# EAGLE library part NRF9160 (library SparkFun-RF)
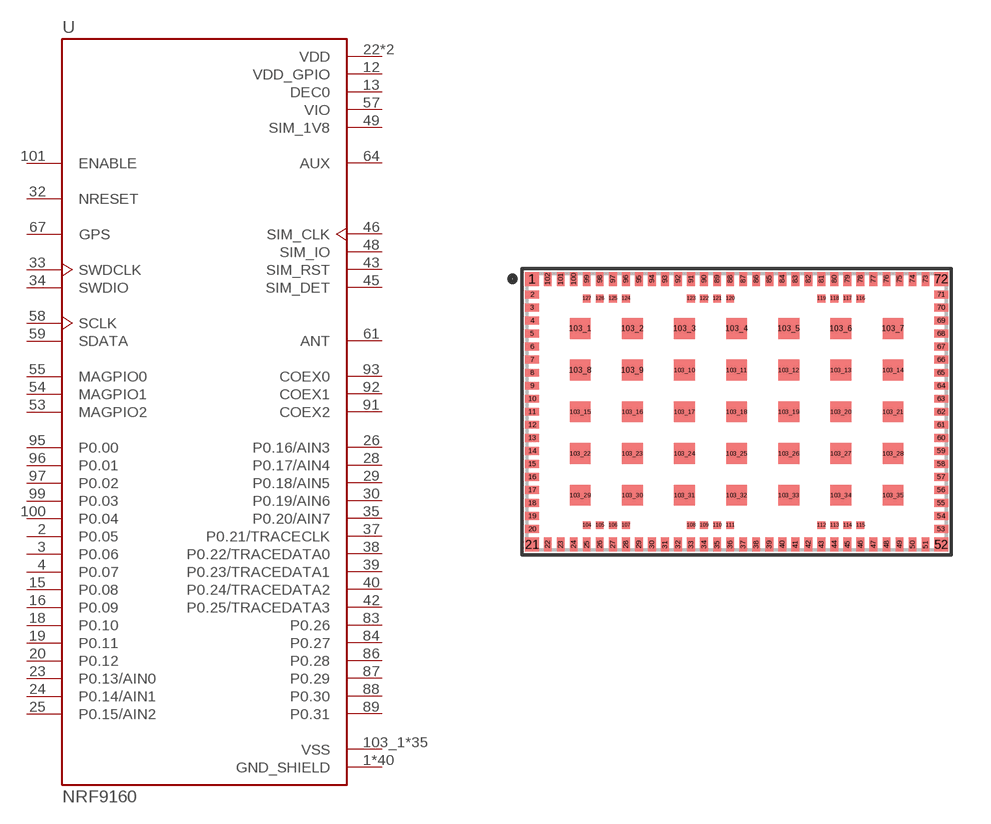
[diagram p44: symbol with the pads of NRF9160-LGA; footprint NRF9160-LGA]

Designator prefix -

## NRF9160 (PROD_ID: IC-15418; VALUE: NRF9160-SICA-R)  [NRF9160-LGA]
1  GND_SHIELD  pwr
2  P0.05
3  P0.06
4  P0.07
5  GND_SHIELD  pwr
6  GND_SHIELD  pwr
7  GND_SHIELD  pwr
8  GND_SHIELD  pwr
9  GND_SHIELD  pwr
11  GND_SHIELD  pwr
12  VDD_GPIO  pwr
13  DEC0  pwr
14  GND_SHIELD  pwr
15  P0.08
16  P0.09
17  GND_SHIELD  pwr
18  P0.10
19  P0.11
20  P0.12
21  GND_SHIELD  pwr
22  VDD  pwr
23  P0.13/AIN0
24  P0.14/AIN1
25  P0.15/AIN2
26  P0.16/AIN3
27  GND_SHIELD  pwr
28  P0.17/AIN4
29  P0.18/AIN5
30  P0.19/AIN6
31  GND_SHIELD  pwr
32  NRESET  in
33  SWDCLK  in
34  SWDIO
35  P0.20/AIN7
36  GND_SHIELD  pwr
37  P0.21/TRACECLK
38  P0.22/TRACEDATA0
39  P0.23/TRACEDATA1
40  P0.24/TRACEDATA2
41  GND_SHIELD  pwr
42  P0.25/TRACEDATA3
43  SIM_RST
44  GND_SHIELD  pwr
45  SIM_DET
46  SIM_CLK
47  GND_SHIELD  pwr
48  SIM_IO
49  SIM_1V8  pwr
50  GND_SHIELD  pwr
52  GND_SHIELD  pwr
53  MAGPIO2
54  MAGPIO1
55  MAGPIO0
56  GND_SHIELD  pwr
57  VIO  pwr
58  SCLK
59  SDATA
60  GND_SHIELD  pwr
61  ANT
62  GND_SHIELD  pwr
63  GND_SHIELD  pwr
64  AUX  out
65  GND_SHIELD  pwr
66  GND_SHIELD  pwr
67  GPS  in
68  GND_SHIELD  pwr
69  GND_SHIELD  pwr
72  GND_SHIELD  pwr
74  GND_SHIELD  pwr
75  GND_SHIELD  pwr
76  GND_SHIELD  pwr
77  GND_SHIELD  pwr
78  GND_SHIELD  pwr
79  GND_SHIELD  pwr
80  GND_SHIELD  pwr
81  GND_SHIELD  pwr
82  GND_SHIELD  pwr
83  P0.26
84  P0.27
85  GND_SHIELD  pwr
86  P0.28
87  P0.29
88  P0.30
89  P0.31
90  GND_SHIELD  pwr
91  COEX2
92  COEX1
93  COEX0
94  GND_SHIELD  pwr
95  P0.00
96  P0.01
97  P0.02
98  GND_SHIELD  pwr
99  P0.03
100  P0.04
101  ENABLE  in
102  VDD  pwr
103_1  VSS  pwr
103_2  VSS  pwr
103_3  VSS  pwr
103_4  VSS  pwr
103_5  VSS  pwr
103_6  VSS  pwr
103_7  VSS  pwr
103_8  VSS  pwr
103_9  VSS  pwr
103_10  VSS  pwr
103_11  VSS  pwr
103_12  VSS  pwr
103_13  VSS  pwr
103_14  VSS  pwr
103_15  VSS  pwr
103_16  VSS  pwr
103_17  VSS  pwr
103_18  VSS  pwr
103_19  VSS  pwr
103_20  VSS  pwr
103_21  VSS  pwr
103_22  VSS  pwr
103_23  VSS  pwr
103_24  VSS  pwr
103_25  VSS  pwr
103_26  VSS  pwr
103_27  VSS  pwr
103_28  VSS  pwr
103_29  VSS  pwr
103_30  VSS  pwr
103_31  VSS  pwr
103_32  VSS  pwr
103_33  VSS  pwr
103_34  VSS  pwr
103_35  VSS  pwr

## Footprint NRF9160-LGA (pad centres in mm)
smd 0.54 x 0.54: 1 -7.845,5.095; 21 -7.845,-5.095; 52 7.845,-5.095; 72 7.845,5.095
smd 0.54 x 0.3: 2 -7.845,4.5; 3 -7.845,4; 4 -7.845,3.5; 5 -7.845,3; 6 -7.845,2.5; 7 -7.845,2; 8 -7.845,1.5; 9 -7.845,1; 10 -7.845,0.5; 11 -7.845,0; 12 -7.845,-0.5; 13 -7.845,-1; 14 -7.845,-1.5; 15 -7.845,-2; 16 -7.845,-2.5; 17 -7.845,-3; 18 -7.845,-3.5; 19 -7.845,-4; 20 -7.845,-4.5; 53 7.845,-4.5; 54 7.845,-4; 55 7.845,-3.5; 56 7.845,-3; 57 7.845,-2.5; 58 7.845,-2; 59 7.845,-1.5; 60 7.845,-1; 61 7.845,-0.5; 62 7.845,0; 63 7.845,0.5; 64 7.845,1; 65 7.845,1.5; 66 7.845,2; 67 7.845,2.5; 68 7.845,3; 69 7.845,3.5; 70 7.845,4; 71 7.845,4.5
smd 0.3 x 0.54: 22 -7.25,-5.095; 23 -6.75,-5.095; 24 -6.25,-5.095; 25 -5.75,-5.095; 26 -5.25,-5.095; 27 -4.75,-5.095; 28 -4.25,-5.095; 29 -3.75,-5.095; 30 -3.25,-5.095; 31 -2.75,-5.095; 32 -2.25,-5.095; 33 -1.75,-5.095; 34 -1.25,-5.095; 35 -0.75,-5.095; 36 -0.25,-5.095; 37 0.25,-5.095; 38 0.75,-5.095; 39 1.25,-5.095; 40 1.75,-5.095; 41 2.25,-5.095; 42 2.75,-5.095; 43 3.25,-5.095; 44 3.75,-5.095; 45 4.25,-5.095; 46 4.75,-5.095; 47 5.25,-5.095; 48 5.75,-5.095; 49 6.25,-5.095; 50 6.75,-5.095; 51 7.25,-5.095; 73 7.25,5.095; 74 6.75,5.095; 75 6.25,5.095; 76 5.75,5.095; 77 5.25,5.095; 78 4.75,5.095; 79 4.25,5.095; 80 3.75,5.095; 81 3.25,5.095; 82 2.75,5.095; 83 2.25,5.095; 84 1.75,5.095; 85 1.25,5.095; 86 0.75,5.095; 87 0.25,5.095; 88 -0.25,5.095; 89 -0.75,5.095; 90 -1.25,5.095; 91 -1.75,5.095; 92 -2.25,5.095; 93 -2.75,5.095; 94 -3.25,5.095; 95 -3.75,5.095; 96 -4.25,5.095; 97 -4.75,5.095; 98 -5.25,5.095; 99 -5.75,5.095; 100 -6.25,5.095; 101 -6.75,5.095; 102 -7.25,5.095
smd 0.8 x 0.8: 103_1 -6,3.2; 103_2 -4,3.2; 103_3 -2,3.2; 103_4 0,3.2; 103_5 2,3.2; 103_6 4,3.2; 103_7 6,3.2; 103_8 -6,1.6; 103_9 -4,1.6; 103_10 -2,1.6; 103_11 0,1.6; 103_12 2,1.6; 103_13 4,1.6; 103_14 6,1.6; 103_15 -6,0; 103_16 -4,0; 103_17 -2,0; 103_18 0,0; 103_19 2,0; 103_20 4,0; 103_21 6,0; 103_22 -6,-1.6; 103_23 -4,-1.6; 103_24 -2,-1.6; 103_25 0,-1.6; 103_26 2,-1.6; 103_27 4,-1.6; 103_28 6,-1.6; 103_29 -6,-3.2; 103_30 -4,-3.2; 103_31 -2,-3.2; 103_32 0,-3.2; 103_33 2,-3.2; 103_34 4,-3.2; 103_35 6,-3.2
smd 0.3 x 0.3: 104 -5.75,-4.35; 105 -5.25,-4.35; 106 -4.75,-4.35; 107 -4.25,-4.35; 108 -1.75,-4.35; 109 -1.25,-4.35; 110 -0.75,-4.35; 111 -0.25,-4.35; 112 3.25,-4.35; 113 3.75,-4.35; 114 4.25,-4.35; 115 4.75,-4.35; 116 4.75,4.35; 117 4.25,4.35; 118 3.75,4.35; 119 3.25,4.35; 120 -0.25,4.35; 121 -0.75,4.35; 122 -1.25,4.35; 123 -1.75,4.35; 124 -4.25,4.35; 125 -4.75,4.35; 126 -5.25,4.35; 127 -5.75,4.35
